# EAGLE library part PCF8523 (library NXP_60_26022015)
The PCF8523 is a CMOS Real-Time Clock (RTC) and calendar optimized for low power consumption. Data is transferred serially via an I2C-bus with a maximum data rate of 1000 kbit/s. Alarm and timer functions are available with the possibility to generate a wake-up signal on an interrupt pin. An offset register allows fine-tuning of the clock. The PCF8523 has a backup battery switch-over circuit, which detects power failures and automatically switches to the battery supply when a power failure occurs. AAL Eindhoven MK
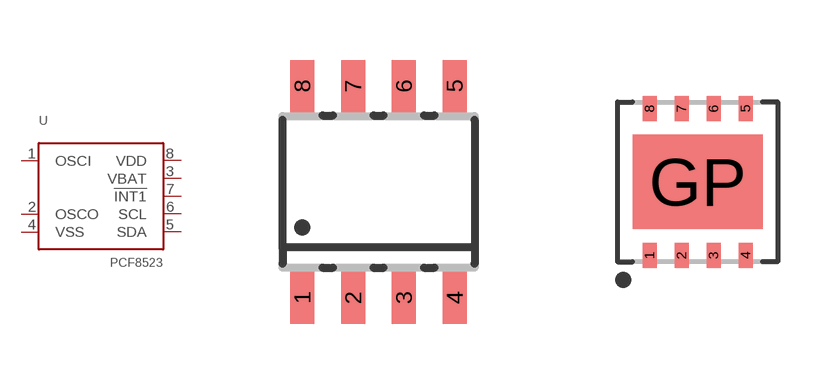
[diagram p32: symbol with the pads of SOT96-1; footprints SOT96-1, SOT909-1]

Designator prefix U

## PCF8523T  [SOT96-1]
1  OSCI  pas
2  OSCO  pas
3  VBAT  pwr
4  VSS  pwr
5  SDA
6  SCL  in
7  !INT1  out
8  VDD  pwr

## PCF8523TK  [SOT909-1]
Pads as for SOT96-1

## Footprint SOT96-1 (pad centres in mm)
SOT96-1 SO8: plastic small outline package; 8 leads; body width 3.9 mm JEDEC: MS-012 IEC: 076E03
smd 0.6 x 1.3: 1 -1.905,-2.65; 2 -0.635,-2.65; 3 0.635,-2.65; 4 1.905,-2.65; 5 1.905,2.65; 6 0.635,2.65; 7 -0.635,2.65; 8 -1.905,2.65

## Footprint SOT909-1 (pad centres in mm)
SOT909-1 HVSON8: plastic thermal enhanced very thin small outline package; no leads; 8 terminals; body 4 x 4 x 0.85 mm JEDEC: -- IEC: MO-229 JEITA: --
smd 0.35 x 0.625: 1 -1.2,-1.837; 2 -0.4,-1.837; 3 0.4,-1.837; 4 1.2,-1.837; 5 1.2,1.837; 6 0.4,1.837; 7 -0.4,1.837; 8 -1.2,1.837
smd 3.25 x 2.35: GP 0,0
